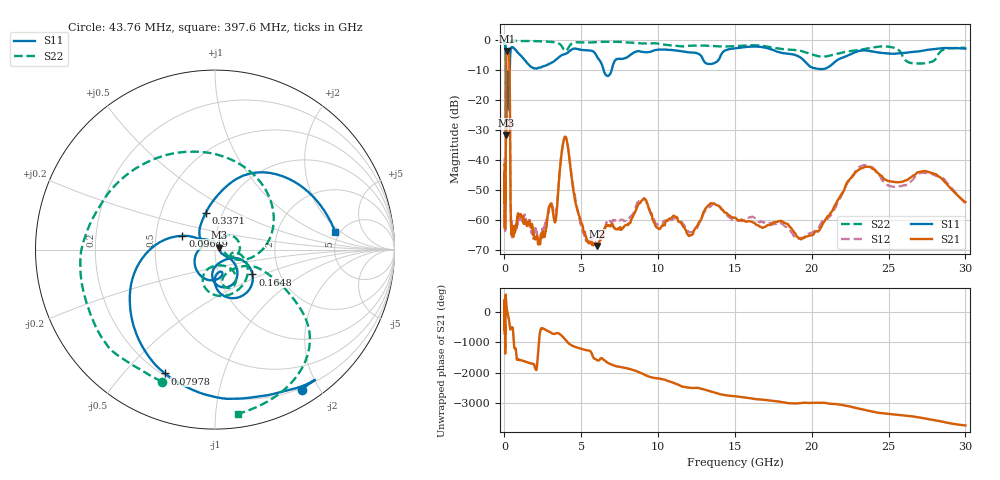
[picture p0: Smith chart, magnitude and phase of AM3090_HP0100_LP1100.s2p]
! Date/Time: Thu, Feb 28, 2019 1:58 PM
! Network Analyzer: Agilent Technologies E8364B Rev: A.07.50.67
! Sweep from 0.010 to 30.000 GHz, 1601 Points, Sweep Type: LOG
! Power Supply: 5.023 V, 0.002 A
# Hz S DB R 50
!freq MagS11 AngS11 MagS21 AngS21 MagS12 AngS12 MagS22 AngS22
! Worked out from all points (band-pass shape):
!   1601 points, 10 MHz to 30 GHz, reference 50 ohm
!   highest |S21| = -3.67 dB at 159.9 MHz (marker M1); lowest = -68.7 dB at 6.049 GHz (marker M2)
!   |S21| within 3 dB of the highest: 106.7 MHz to 320.3 MHz (213.6 MHz wide, 100 % of centre)
!   lowest |S11| = -31.7 dB at 103.5 MHz (marker M3), VSWR 1.05, Z = 52.4 + j1.18 ohm
!   |S11| at or under -10 dB: 94.44 MHz to 349.5 MHz (255.1 MHz wide, 115 % of centre); 6.455 GHz to 6.977 GHz (521.4 MHz wide, 7.76 % of centre)
!   |S22| runs from -29.4 to -0.1 dB; largest |S21 - S12| = 0.012
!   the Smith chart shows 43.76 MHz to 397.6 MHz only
!   S11 on the Smith chart (normalised r, x): 43.76 MHz: 0.18, -1.78; 79.78 MHz: 0.21, -0.65; 96.49 MHz: 0.68, +0.11; 164.8 MHz: 1.45, -0.43; 337.1 MHz: 0.83, +0.36; 397.6 MHz: 4.59, +1.63
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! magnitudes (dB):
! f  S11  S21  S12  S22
! 10 MHz  -0.3  -41.4  -39.3  -0.7
! 38.04 MHz  -0.5  -59.2  -59.7  -1.6
! 43.76 MHz  -0.8  -59.4  -59.4  -2.0
! 79.78 MHz  -2.6  -47.8  -50.3  -4.7
! 96.49 MHz  -14.1  -14.1  -14.1  -13.6
! 103.5 MHz  -31.7  -7.8  -7.8  -28.5
! 119.1 MHz  -13.3  -5.0  -5.0  -18.1
! 144.7 MHz  -22.0  -3.8  -3.8  -20.8
! 159.9 MHz  -13.3  -3.7  -3.6  -16.0
! 164.8 MHz  -12.0  -3.7  -3.7  -14.5
! 337.1 MHz  -13.5  -10.0  -10.0  -8.4
! 397.6 MHz  -3.4  -54.1  -53.8  -0.7
! 550.5 MHz  -2.5  -65.1  -62.3  -0.2
! 2.084 GHz  -9.5  -65.7  -64.1  -0.4
! 3.318 GHz  -6.7  -60.6  -58.2  -0.8
! 3.953 GHz  -4.7  -32.3  -32.2  -3.6
! 5.103 GHz  -3.3  -62.2  -64.2  -0.8
! 6.049 GHz  -5.8  -68.7  -68.3  -0.7
! 7.926 GHz  -5.9  -61.7  -60.1  -0.8
! 19.51 GHz  -6.9  -66.0  -65.7  -3.9
! 23.48 GHz  -3.4  -42.2  -41.8  -2.9
! 30 GHz  -2.8  -54.1  -54.6  -2.6
